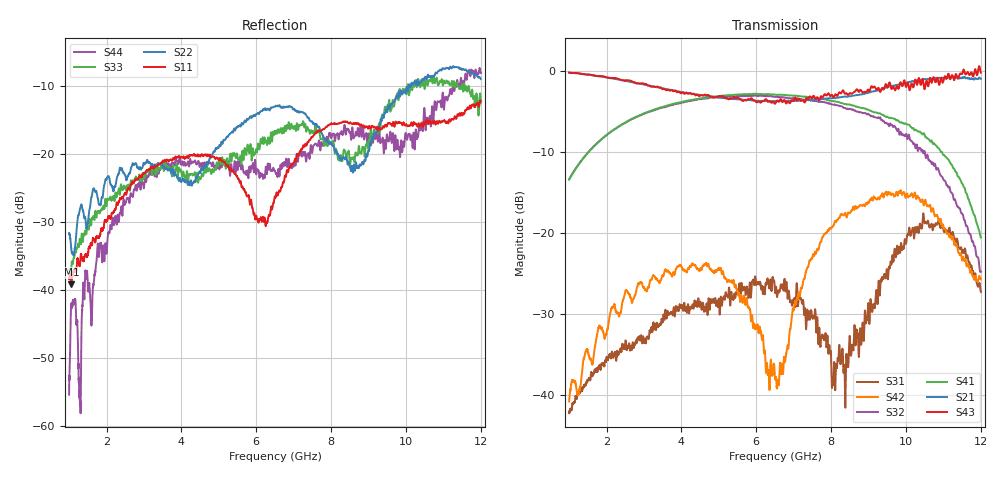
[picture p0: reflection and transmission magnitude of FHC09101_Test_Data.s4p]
!Keysight Technologies,N5227B,US57180409,A.15.40.08
!Date: Thursday, February 01, 2024 13:30:40
!Correction: S11(C  4-Port  )
!S12(C  4-Port  )
!S13(C  4-Port  )
!S14(C  4-Port  )
!S21(C  4-Port  )
!S22(C  4-Port  )
!S23(C  4-Port  )
!S24(C  4-Port  )
!S31(C  4-Port  )
!S32(C  4-Port  )
!S33(C  4-Port  )
!S34(C  4-Port  )
!S41(C  4-Port  )
!S42(C  4-Port  )
!S43(C  4-Port  )
!S44(C  4-Port  )
!S4P File: Measurements: <S11,S12,S13,S14>,
!<S21,S22,S23,S24>,
!<S31,S32,S33,S34>,
!<S41,S42,S43,S44>:
# Hz S  dB  R 50
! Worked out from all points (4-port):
!   6401 points, 1 GHz to 12 GHz, reference 50 ohm
!   strongest paths, dB at 1 GHz, 3.75 GHz, 6.5 GHz, 9.25 GHz, 12 GHz:
!     S43: -0.2, -2.3, -4.0, -2.1, -0.2
!     S21: -0.2, -2.3, -3.7, -2.4, -0.9
!     S41: -13.4, -4.1, -2.9, -5.2, -20.6
!     S32: -13.4, -4.1, -3.2, -5.7, -24.8
!     S42: -40.8, -25.4, -37.9, -15.7, -25.7
!     S31: -42.2, -29.8, -27.3, -27.9, -27.3
!   lowest |S11| = -39.2 dB at 1.062 GHz (marker M1), VSWR 1.02, Z = 49.4 + j0.897 ohm
!   |S11| at or under -10 dB: start of sweep to end of sweep
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1e9  -38.39 121.3  -0.18 -45.8  -42.27 34.7  -13.41 44.6
     -0.17 -45.8  -31.65 137.0  -13.37 42.8  -40.81 29.9
     -42.20 34.3  -13.36 42.8  -37.69 156.7  -0.18 -44.7
     -13.39 44.6  -40.81 30.3  -0.18 -44.7  -55.35 -35.1
1.061875e9  -39.15 124.5  -0.21 -48.6  -41.90 32.0  -12.90 41.8
            -0.20 -48.6  -34.21 143.4  -12.86 39.9  -38.54 36.6
            -41.80 32.0  -12.86 40.0  -36.53 158.1  -0.22 -47.7
            -12.90 41.8  -38.55 36.5  -0.23 -47.8  -42.01 -34.5
3.554062e9  -20.96 90.5  -2.22 -159.6  -30.33 -94.6  -4.34 -68.9
            -2.15 -159.7  -22.16 66.8  -4.41 -75.1  -24.63 -130.2
            -30.34 -94.0  -4.47 -74.8  -20.97 84.2  -2.24 -155.4
            -4.33 -68.8  -24.69 -130.2  -2.24 -155.7  -21.52 113.0
6.237031e9  -30.11 86.1  -3.80 87.0  -26.95 120.8  -2.88 179.1
            -3.67 86.8  -13.31 74.7  -2.87 166.3  -34.76 29.1
            -26.97 121.2  -3.04 166.8  -18.11 84.5  -3.58 93.4
            -2.84 179.1  -34.84 29.3  -3.50 93.1  -22.84 -74.3
9.117656e9  -16.05 76.4  -2.71 -33.5  -28.98 111.7  -5.02 59.4
            -2.52 -34.7  -17.88 106.2  -5.27 37.0  -15.75 81.5
            -29.10 112.1  -5.59 38.4  -17.63 105.9  -2.18 -24.8
            -5.01 59.4  -15.95 82.8  -2.03 -24.9  -18.40 46.6
1.047891e10  -15.34 86.7  -1.35 -96.4  -18.40 43.6  -7.97 0.7
             -1.01 -99.0  -9.19 79.8  -9.91 -29.7  -16.51 2.7
             -18.18 43.0  -10.01 -27.7  -9.63 75.2  -1.96 -79.3
             -7.70 -0.6  -16.58 4.2  -1.90 -80.0  -13.59 -110.6
1.2e10  -12.32 86.1  -1.21 -166.3  -26.70 -34.0  -20.23 -53.5
        -0.94 -172.5  -9.03 28.6  -23.94 -76.4  -25.09 -20.5
        -27.27 -34.3  -24.77 -70.3  -12.51 24.0  -0.46 -152.5
        -20.56 -54.9  -25.68 -15.8  -0.19 -153.7  -8.15 106.3
